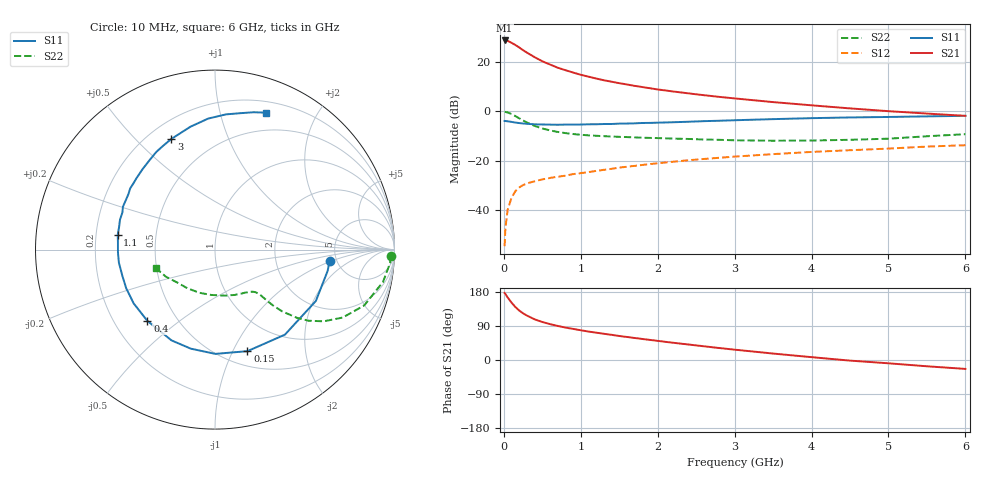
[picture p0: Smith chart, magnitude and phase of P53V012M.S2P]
! SIEMENS Small Signal Semiconductors
! BFP183
! Si NPN RF Bipolar Junction Transistor in SOT143
! VCE = 3 V  IC = 12 mA
! Common Emitter S-Parameters:  March  1996
# GHz  S  MA  R  50
!  f  S11  S21  S12  S22
! GHz  MAG  ANG  MAG  ANG  MAG  ANG  MAG  ANG
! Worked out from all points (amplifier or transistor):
!   36 points, 10 MHz to 6 GHz, reference 50 ohm
!   highest |S21| = 28.9 dB at 10 MHz (marker M1)
!   |S21| within 3 dB of that: start of sweep to 206.4 MHz
!   unconditionally stable (mu >= 1): 1.045 GHz to 5.493 GHz
!   at 250 MHz: K = 0.36, MSG = 27.5 dB, |S12| = -30.0 dB
!   at 1.4 GHz: K = 1.11, MAG = 15.8 dB, |S12| = -23.4 dB
!   at 6 GHz: K = 0.95, MSG = 6.0 dB, |S12| = -13.8 dB
!   S11 on the Smith chart (normalised r, x): 10 MHz: 4.38, -0.92; 150 MHz: 0.65, -1.14; 400 MHz: 0.34, -0.39; 1.1 GHz: 0.29, +0.07; 3 GHz: 0.29, +0.64; 6 GHz: 0.31, +1.40
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0.01  0.6416 -5.5  28 176.9  0.0018 89.3  0.9815 -2.1
0.02  0.6387 -10.7  28 174.2  0.0041 81.7  0.9785 -4.4
0.05  0.6307 -27.0  27.47 164.9  0.01 80.2  0.9533 -10.9
0.1  0.6134 -50.6  25.08 151.5  0.0175 66.5  0.8878 -20.5
0.15  0.594 -72.3  22.66 139.8  0.0237 60.4  0.8062 -28.0
0.2  0.581 -89.8  20.16 130.5  0.0282 54.9  0.7257 -33.4
0.25  0.5682 -103.7  17.73 123.1  0.0316 50.8  0.6557 -37.2
0.3  0.5609 -115.6  15.85 117.2  0.0342 48.0  0.5965 -39.7
0.4  0.5474 -133.5  12.79 107.3  0.0378 44.8  0.5083 -42.6
0.5  0.5433 -146.5  10.55 100.3  0.0413 43.1  0.45 -43.9
0.6  0.5396 -156.5  9.061 94.7  0.0442 43.5  0.4112 -44.4
0.7  0.5365 -164.5  7.801 89.9  0.0467 43.7  0.3829 -44.7
0.9  0.5409 -178.2  6.221 82.1  0.0529 44.7  0.3474 -45.3
1.1  0.5483 171.3  5.121 75.1  0.0583 45.4  0.3263 -46.6
1.5  0.5658 155.0  3.775 63.3  0.0718 46.0  0.3044 -50.7
1.8  0.5827 144.2  3.147 55.5  0.0812 45.9  0.2921 -55.2
2.2  0.6034 131.9  2.557 45.5  0.0946 44.4  0.2802 -62.4
3  0.6628 111.5  1.846 27.3  0.1203 39.5  0.2589 -81.0
3.5  0.6982 101.3  1.553 17.0  0.1352 36.0  0.2536 -94.7
4.5  0.7558 85.4  1.156 -1.6  0.1625 28.1  0.2648 -125.6
5.5  0.795 74.3  0.907 -16.6  0.1927 20.9  0.3126 -151.1
6  0.8149 69.4  0.815 -23.5  0.2053 16.6  0.3446 -162.5
